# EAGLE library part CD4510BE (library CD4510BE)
CD4510BE, 4-stage BCD Counter, Decade Up/Down Counter, Bi-Directional, 3 18 V, 16-Pin PDIP Source: Datasheet
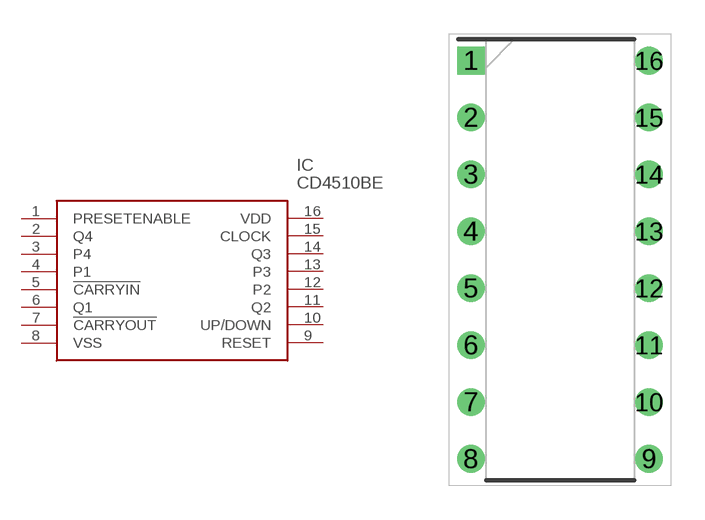
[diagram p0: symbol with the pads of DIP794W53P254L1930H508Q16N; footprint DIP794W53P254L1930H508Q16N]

Designator prefix IC

## CD4510BE (Arrow_Part_Number: CD4510BE; Arrow_Price-Stock: https://www.arrow.com/en/products/cd4510be/texas-instruments?region=nac; Description: CD4510BE, 4-stage BCD Counter, Decade Up/Down Counter, Bi-Directional, 3 18 V, 16-Pin PDIP; Height: 5.08mm; Manufacturer_Name: Texas Instruments; Manufacturer_Part_Number: CD4510BE; Mouser_Part_Number: 595-CD4510BE; Mouser_Price-Stock: https://www.mouser.co.uk/ProductDetail/Texas-Instruments/CD4510BE?qs=YxwvVplHM%2FkYHJ644QIwGQ%3D%3D)  [DIP794W53P254L1930H508Q16N]
1  PRESETENABLE
2  Q4
3  P4
4  P1
5  !CARRYIN  in
6  Q1
7  !CARRYOUT  out
8  VSS  pwr
9  RESET
10  UP/DOWN
11  Q2
12  P2
13  P3
14  Q3
15  CLOCK  in
16  VDD  pwr

## Footprint DIP794W53P254L1930H508Q16N (pad centres in mm)
N (R-PDIP-T16)
drill 0.73 pad 1.13 square: 1 -3.97,8.89
drill 0.73 pad 1.13: 2 -3.97,6.35; 3 -3.97,3.81; 4 -3.97,1.27; 5 -3.97,-1.27; 6 -3.97,-3.81; 7 -3.97,-6.35; 8 -3.97,-8.89; 9 3.97,-8.89; 10 3.97,-6.35; 11 3.97,-3.81; 12 3.97,-1.27; 13 3.97,1.27; 14 3.97,3.81; 15 3.97,6.35; 16 3.97,8.89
